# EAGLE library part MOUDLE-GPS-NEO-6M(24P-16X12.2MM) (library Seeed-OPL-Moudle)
317050000
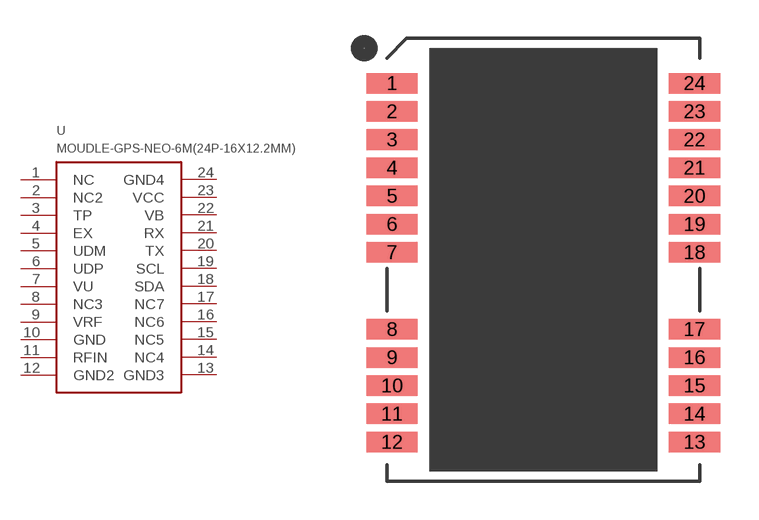
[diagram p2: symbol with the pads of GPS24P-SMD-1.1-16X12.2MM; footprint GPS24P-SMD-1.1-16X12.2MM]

Designator prefix U

## MOUDLE-GPS-NEO-6M(24P-16X12.2MM) (MPN: NEO-6M-GPS; VALUE: NEO-6M-GPS(24p-16x12.2x2.4mm))  [GPS24P-SMD-1.1-16X12.2MM]
1  NC
2  NC2
3  TP
4  EX
5  UDM
6  UDP
7  VU
8  NC3
9  VRF
10  GND
11  RFIN
12  GND2
13  GND3
14  NC4
15  NC5
16  NC6
17  NC7
18  SDA
19  SCL
20  TX
21  RX
22  VB
23  VCC
24  GND4

## Footprint GPS24P-SMD-1.1-16X12.2MM (pad centres in mm)
smd 2 x 0.8: 1 -5.904,6.888; 2 -5.904,5.788; 3 -5.904,4.688; 4 -5.904,3.588; 5 -5.904,2.488; 6 -5.904,1.388; 7 -5.904,0.288; 8 -5.904,-2.712; 9 -5.904,-3.812; 10 -5.904,-4.912; 11 -5.904,-6.012; 12 -5.904,-7.112; 13 5.896,-7.112; 14 5.896,-6.012; 15 5.896,-4.912; 16 5.896,-3.812; 17 5.896,-2.712; 18 5.896,0.288; 19 5.896,1.388; 20 5.896,2.488; 21 5.896,3.588; 22 5.896,4.688; 23 5.896,5.788; 24 5.896,6.888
